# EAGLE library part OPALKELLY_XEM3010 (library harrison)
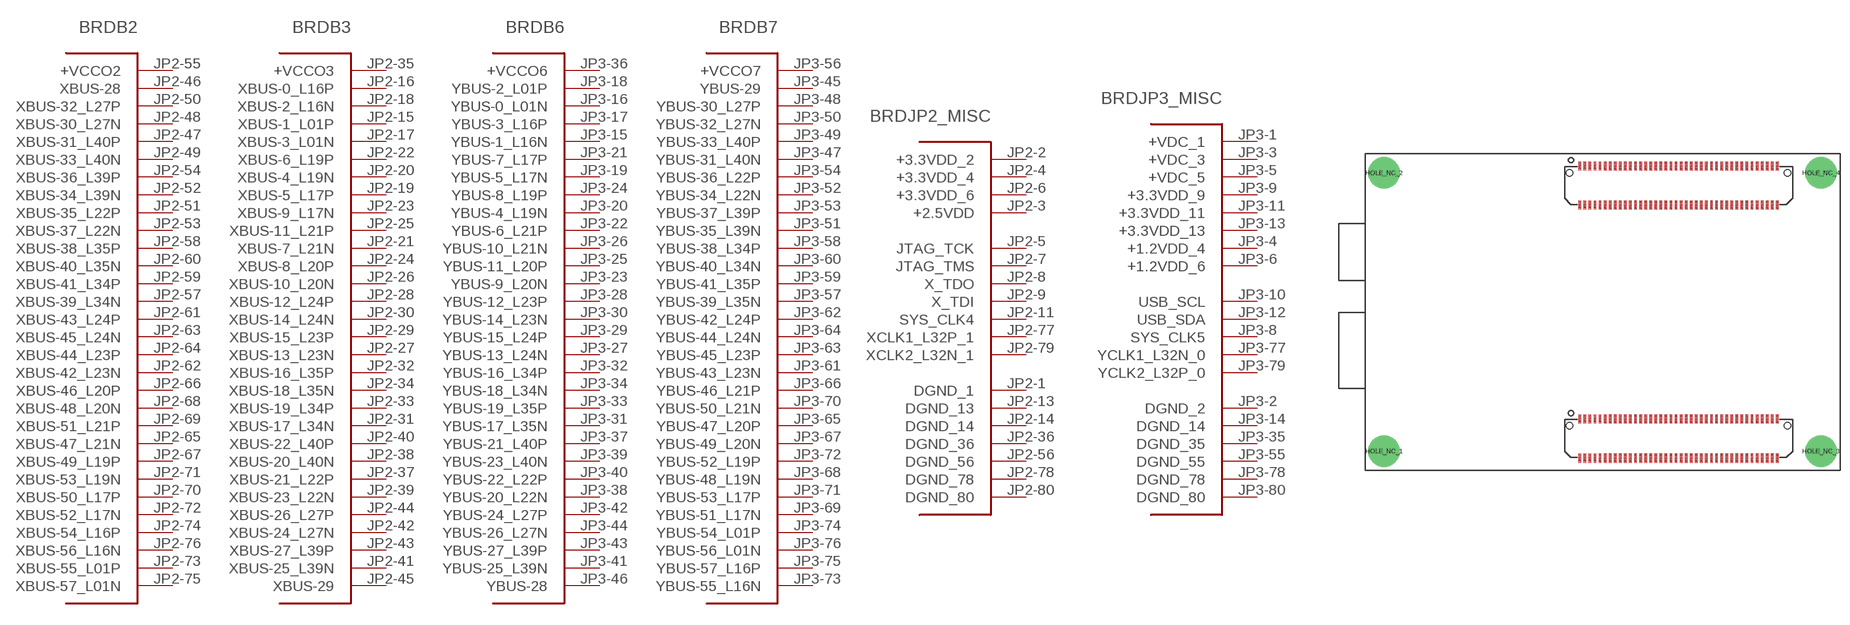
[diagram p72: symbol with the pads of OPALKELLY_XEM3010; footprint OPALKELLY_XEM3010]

Designator prefix BRD; gates B2=XEM3010_JP2_BANK2 B3=XEM3010_JP2_BANK3 B6=XEM3010_JP3_BANK6 B7=XEM3010_JP3_BANK7 JP2_MISC=XEM3010_JP2_MISC JP3_MISC=XEM3010_JP3_MISC

## OPALKELLY_XEM3010  [OPALKELLY_XEM3010]
JP2-1  JP2_MISC:DGND_1  pwr
JP2-2  JP2_MISC:+3.3VDD_2  pwr
JP2-3  JP2_MISC:+2.5VDD  pwr
JP2-4  JP2_MISC:+3.3VDD_4  pwr
JP2-5  JP2_MISC:JTAG_TCK
JP2-6  JP2_MISC:+3.3VDD_6  pwr
JP2-7  JP2_MISC:JTAG_TMS
JP2-8  JP2_MISC:X_TDO
JP2-9  JP2_MISC:X_TDI
JP2-11  JP2_MISC:SYS_CLK4  out
JP2-13  JP2_MISC:DGND_13  pwr
JP2-14  JP2_MISC:DGND_14  pwr
JP2-15  B3:XBUS-1_L01P
JP2-16  B3:XBUS-0_L16P
JP2-17  B3:XBUS-3_L01N
JP2-18  B3:XBUS-2_L16N
JP2-19  B3:XBUS-5_L17P
JP2-20  B3:XBUS-4_L19N
JP2-21  B3:XBUS-7_L21N
JP2-22  B3:XBUS-6_L19P
JP2-23  B3:XBUS-9_L17N
JP2-24  B3:XBUS-8_L20P
JP2-25  B3:XBUS-11_L21P
JP2-26  B3:XBUS-10_L20N
JP2-27  B3:XBUS-13_L23N
JP2-28  B3:XBUS-12_L24P
JP2-29  B3:XBUS-15_L23P
JP2-30  B3:XBUS-14_L24N
JP2-31  B3:XBUS-17_L34N
JP2-32  B3:XBUS-16_L35P
JP2-33  B3:XBUS-19_L34P
JP2-34  B3:XBUS-18_L35N
JP2-35  B3:+VCCO3  pwr
JP2-36  JP2_MISC:DGND_36  pwr
JP2-37  B3:XBUS-21_L22P
JP2-38  B3:XBUS-20_L40N
JP2-39  B3:XBUS-23_L22N
JP2-40  B3:XBUS-22_L40P
JP2-41  B3:XBUS-25_L39N
JP2-42  B3:XBUS-24_L27N
JP2-43  B3:XBUS-27_L39P
JP2-44  B3:XBUS-26_L27P
JP2-45  B3:XBUS-29
JP2-46  B2:XBUS-28
JP2-47  B2:XBUS-31_L40P
JP2-48  B2:XBUS-30_L27N
JP2-49  B2:XBUS-33_L40N
JP2-50  B2:XBUS-32_L27P
JP2-51  B2:XBUS-35_L22P
JP2-52  B2:XBUS-34_L39N
JP2-53  B2:XBUS-37_L22N
JP2-54  B2:XBUS-36_L39P
JP2-55  B2:+VCCO2  pwr
JP2-56  JP2_MISC:DGND_56  pwr
JP2-57  B2:XBUS-39_L34N
JP2-58  B2:XBUS-38_L35P
JP2-59  B2:XBUS-41_L34P
JP2-60  B2:XBUS-40_L35N
JP2-61  B2:XBUS-43_L24P
JP2-62  B2:XBUS-42_L23N
JP2-63  B2:XBUS-45_L24N
JP2-64  B2:XBUS-44_L23P
JP2-65  B2:XBUS-47_L21N
JP2-66  B2:XBUS-46_L20P
JP2-67  B2:XBUS-49_L19P
JP2-68  B2:XBUS-48_L20N
JP2-69  B2:XBUS-51_L21P
JP2-70  B2:XBUS-50_L17P
JP2-71  B2:XBUS-53_L19N
JP2-72  B2:XBUS-52_L17N
JP2-73  B2:XBUS-55_L01P
JP2-74  B2:XBUS-54_L16P
JP2-75  B2:XBUS-57_L01N
JP2-76  B2:XBUS-56_L16N
JP2-77  JP2_MISC:XCLK1_L32P_1  in
JP2-78  JP2_MISC:DGND_78  pwr
JP2-79  JP2_MISC:XCLK2_L32N_1  in
JP2-80  JP2_MISC:DGND_80  pwr
JP3-1  JP3_MISC:+VDC_1  pwr
JP3-2  JP3_MISC:DGND_2  pwr
JP3-3  JP3_MISC:+VDC_3  pwr
JP3-4  JP3_MISC:+1.2VDD_4  pwr
JP3-5  JP3_MISC:+VDC_5  pwr
JP3-6  JP3_MISC:+1.2VDD_6  pwr
JP3-8  JP3_MISC:SYS_CLK5  out
JP3-9  JP3_MISC:+3.3VDD_9  pwr
JP3-10  JP3_MISC:USB_SCL
JP3-11  JP3_MISC:+3.3VDD_11  pwr
JP3-12  JP3_MISC:USB_SDA
JP3-13  JP3_MISC:+3.3VDD_13  pwr
JP3-14  JP3_MISC:DGND_14  pwr
JP3-15  B6:YBUS-1_L16N
JP3-16  B6:YBUS-0_L01N
JP3-17  B6:YBUS-3_L16P
JP3-18  B6:YBUS-2_L01P
JP3-19  B6:YBUS-5_L17N
JP3-20  B6:YBUS-4_L19N
JP3-21  B6:YBUS-7_L17P
JP3-22  B6:YBUS-6_L21P
JP3-23  B6:YBUS-9_L20N
JP3-24  B6:YBUS-8_L19P
JP3-25  B6:YBUS-11_L20P
JP3-26  B6:YBUS-10_L21N
JP3-27  B6:YBUS-13_L24N
JP3-28  B6:YBUS-12_L23P
JP3-29  B6:YBUS-15_L24P
JP3-30  B6:YBUS-14_L23N
JP3-31  B6:YBUS-17_L35N
JP3-32  B6:YBUS-16_L34P
JP3-33  B6:YBUS-19_L35P
JP3-34  B6:YBUS-18_L34N
JP3-35  JP3_MISC:DGND_35  pwr
JP3-36  B6:+VCCO6  pwr
JP3-37  B6:YBUS-21_L40P
JP3-38  B6:YBUS-20_L22N
JP3-39  B6:YBUS-23_L40N
JP3-40  B6:YBUS-22_L22P
JP3-41  B6:YBUS-25_L39N
JP3-42  B6:YBUS-24_L27P
JP3-43  B6:YBUS-27_L39P
JP3-44  B6:YBUS-26_L27N
JP3-45  B7:YBUS-29
JP3-46  B6:YBUS-28
JP3-47  B7:YBUS-31_L40N
JP3-48  B7:YBUS-30_L27P
JP3-49  B7:YBUS-33_L40P
JP3-50  B7:YBUS-32_L27N
JP3-51  B7:YBUS-35_L39N
JP3-52  B7:YBUS-34_L22N
JP3-53  B7:YBUS-37_L39P
JP3-54  B7:YBUS-36_L22P
JP3-55  JP3_MISC:DGND_55  pwr
JP3-56  B7:+VCCO7  pwr
JP3-57  B7:YBUS-39_L35N
JP3-58  B7:YBUS-38_L34P
JP3-59  B7:YBUS-41_L35P
JP3-60  B7:YBUS-40_L34N
JP3-61  B7:YBUS-43_L23N
JP3-62  B7:YBUS-42_L24P
JP3-63  B7:YBUS-45_L23P
JP3-64  B7:YBUS-44_L24N
JP3-65  B7:YBUS-47_L20P
JP3-66  B7:YBUS-46_L21P
JP3-67  B7:YBUS-49_L20N
JP3-68  B7:YBUS-48_L19N
JP3-69  B7:YBUS-51_L17N
JP3-70  B7:YBUS-50_L21N
JP3-71  B7:YBUS-53_L17P
JP3-72  B7:YBUS-52_L19P
JP3-73  B7:YBUS-55_L16N
JP3-74  B7:YBUS-54_L01P
JP3-75  B7:YBUS-57_L16P
JP3-76  B7:YBUS-56_L01N
JP3-77  JP3_MISC:YCLK1_L32N_0  in
JP3-78  JP3_MISC:DGND_78  pwr
JP3-79  JP3_MISC:YCLK2_L32P_0  in
JP3-80  JP3_MISC:DGND_80  pwr

## Footprint OPALKELLY_XEM3010 (pad centres in mm)
drill 2.5 pad 5: HOLE_NC_1 3,3; HOLE_NC_2 3,47; HOLE_NC_3 72,3; HOLE_NC_4 72,47
smd 0.457 x 1.448: JP2-1 33.9,8.086; JP2-2 33.9,1.914; JP2-3 34.7,8.086; JP2-4 34.7,1.914; JP2-5 35.5,8.086; JP2-6 35.5,1.914; JP2-7 36.3,8.086; JP2-8 36.3,1.914; JP2-9 37.1,8.086; JP2-10 37.1,1.914; JP2-11 37.9,8.086; JP2-12 37.9,1.914; JP2-13 38.7,8.086; JP2-14 38.7,1.914; JP2-15 39.5,8.086; JP2-16 39.5,1.914; JP2-17 40.3,8.086; JP2-18 40.3,1.914; JP2-19 41.1,8.086; JP2-20 41.1,1.914; JP2-21 41.9,8.086; JP2-22 41.9,1.914; JP2-23 42.7,8.086; JP2-24 42.7,1.914; JP2-25 43.5,8.086; JP2-26 43.5,1.914; JP2-27 44.3,8.086; JP2-28 44.3,1.914; JP2-29 45.1,8.086; JP2-30 45.1,1.914; JP2-31 45.9,8.086; JP2-32 45.9,1.914; JP2-33 46.7,8.086; JP2-34 46.7,1.914; JP2-35 47.5,8.086; JP2-36 47.5,1.914; JP2-37 48.3,8.086; JP2-38 48.3,1.914; JP2-39 49.1,8.086; JP2-40 49.1,1.914; JP2-41 49.9,8.086; JP2-42 49.9,1.914; JP2-43 50.7,8.086; JP2-44 50.7,1.914; JP2-45 51.5,8.086; JP2-46 51.5,1.914; JP2-47 52.3,8.086; JP2-48 52.3,1.914; JP2-49 53.1,8.086; JP2-50 53.1,1.914; JP2-51 53.9,8.086; JP2-52 53.9,1.914; JP2-53 54.7,8.086; JP2-54 54.7,1.914; JP2-55 55.5,8.086; JP2-56 55.5,1.914; JP2-57 56.3,8.086; JP2-58 56.3,1.914; JP2-59 57.1,8.086; JP2-60 57.1,1.914; JP2-61 57.9,8.086; JP2-62 57.9,1.914; JP2-63 58.7,8.086; JP2-64 58.7,1.914; JP2-65 59.5,8.086; JP2-66 59.5,1.914; JP2-67 60.3,8.086; JP2-68 60.3,1.914; JP2-69 61.1,8.086; JP2-70 61.1,1.914; JP2-71 61.9,8.086; JP2-72 61.9,1.914; JP2-73 62.7,8.086; JP2-74 62.7,1.914; JP2-75 63.5,8.086; JP2-76 63.5,1.914; JP2-77 64.3,8.086; JP2-78 64.3,1.914; JP2-79 65.1,8.086; JP2-80 65.1,1.914; JP3-1 33.9,48.086; JP3-2 33.9,41.914; JP3-3 34.7,48.086; JP3-4 34.7,41.914; JP3-5 35.5,48.086; JP3-6 35.5,41.914; JP3-7 36.3,48.086; JP3-8 36.3,41.914; JP3-9 37.1,48.086; JP3-10 37.1,41.914; JP3-11 37.9,48.086; JP3-12 37.9,41.914; JP3-13 38.7,48.086; JP3-14 38.7,41.914; JP3-15 39.5,48.086; JP3-16 39.5,41.914; JP3-17 40.3,48.086; JP3-18 40.3,41.914; JP3-19 41.1,48.086; JP3-20 41.1,41.914; JP3-21 41.9,48.086; JP3-22 41.9,41.914; JP3-23 42.7,48.086; JP3-24 42.7,41.914; JP3-25 43.5,48.086; JP3-26 43.5,41.914; JP3-27 44.3,48.086; JP3-28 44.3,41.914; JP3-29 45.1,48.086; JP3-30 45.1,41.914; JP3-31 45.9,48.086; JP3-32 45.9,41.914; JP3-33 46.7,48.086; JP3-34 46.7,41.914; JP3-35 47.5,48.086; JP3-36 47.5,41.914; JP3-37 48.3,48.086; JP3-38 48.3,41.914; JP3-39 49.1,48.086; JP3-40 49.1,41.914; JP3-41 49.9,48.086; JP3-42 49.9,41.914; JP3-43 50.7,48.086; JP3-44 50.7,41.914; JP3-45 51.5,48.086; JP3-46 51.5,41.914; JP3-47 52.3,48.086; JP3-48 52.3,41.914; JP3-49 53.1,48.086; JP3-50 53.1,41.914; JP3-51 53.9,48.086; JP3-52 53.9,41.914; JP3-53 54.7,48.086; JP3-54 54.7,41.914; JP3-55 55.5,48.086; JP3-56 55.5,41.914; JP3-57 56.3,48.086; JP3-58 56.3,41.914; JP3-59 57.1,48.086; JP3-60 57.1,41.914; JP3-61 57.9,48.086; JP3-62 57.9,41.914; JP3-63 58.7,48.086; JP3-64 58.7,41.914; JP3-65 59.5,48.086; JP3-66 59.5,41.914; JP3-67 60.3,48.086; JP3-68 60.3,41.914; JP3-69 61.1,48.086; JP3-70 61.1,41.914; JP3-71 61.9,48.086; JP3-72 61.9,41.914; JP3-73 62.7,48.086; JP3-74 62.7,41.914; JP3-75 63.5,48.086; JP3-76 63.5,41.914; JP3-77 64.3,48.086; JP3-78 64.3,41.914; JP3-79 65.1,48.086; JP3-80 65.1,41.914
hole 1.016 at 32.261,47.032
hole 1.016 at 66.739,47.032
hole 1.016 at 32.261,7.032
hole 1.016 at 66.739,7.032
